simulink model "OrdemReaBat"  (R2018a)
settings: Solver=VariableStepAuto  StartTime=0.0  StopTime=10  RelTol=1e-3
undefined symbols (not defined in the file): bb0aaedc, OrdemReaBat, sdiscope

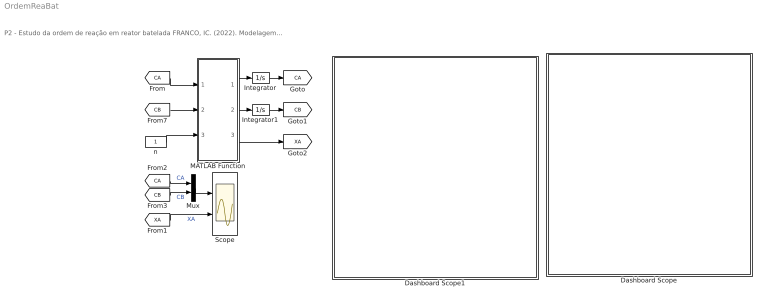
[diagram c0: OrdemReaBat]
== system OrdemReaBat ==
  note: P2 - Estudo da ordem de reação em reator batelada FRANCO, IC. (2022). Modelagem e Simulação: Problemas Típicos da Engenharia Química para Simulação e Análise. NOTAS DE AULA INOVADORAS. The Journal of Engineering and Exact Sciences. Material Complementar.
  Dashboard Scope : Subsystem  DialogController=hmiCreateDDGDialog  IsWebBlock=on  mask(MWDashboardBlock){webBlockId=bb0aaedc-e254-47b2-83d2-97ef23d4ce5b, webBlockType=sdiscope, ShowInitialText=on, HMISrcModelName=OrdemReaBat}
      mask prompts: webBlockId "WebBlock Id"; webBlockType "WebBlock Type"; HMISrcModelName "Source Model"
      mask help: SimulinkHMI:dialogs:HMIScopeDialogDesc
  Dashboard Scope1 : Subsystem  DialogController=hmiCreateDDGDialog  IsWebBlock=on  mask(MWDashboardBlock){webBlockId=9562f2ce-4f72-4572-9857-123cd0054c03, webBlockType=sdiscope, ShowInitialText=on, HMISrcModelName=OrdemReaBat}
      mask prompts: webBlockId "WebBlock Id"; webBlockType "WebBlock Type"; HMISrcModelName "Source Model"
      mask help: SimulinkHMI:dialogs:HMIScopeDialogDesc
  Integrator : Integrator  InitialCondition=1  LowerSaturationLimit=0
  Integrator1 : Integrator  LowerSaturationLimit=0
  MATLAB Function : MATLAB Function  TreatAsAtomicUnit=on
  Mux : Mux  Inputs=2
  Scope : Scope  NumInputPorts=2
  n : Constant
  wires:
  MATLAB Function/1(dCA) -> Integrator/1
  Integrator/1 -> [CA]
  [CA] -> MATLAB Function/1(CA)
  [CA] -> Mux/1  "CA"
  [CB] -> Mux/2  "CB"
  MATLAB Function/3(XA) -> [XA]
  Integrator1/1 -> [CB]
  MATLAB Function/2(dCB) -> Integrator1/1
  [CB] -> MATLAB Function/2(CB)
  n/1 -> MATLAB Function/3(n)
  Mux/1 -> Scope/1
  [XA] -> Scope/2  "XA"

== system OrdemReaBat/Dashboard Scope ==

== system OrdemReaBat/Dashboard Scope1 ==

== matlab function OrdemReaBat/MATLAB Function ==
function [dCA,dCB,XA] = fcn(CA,CB,n)
%% dados do processo
CA0 = 1.00;
k   = 1.30;

%% equações auxiliares
XA=(CA0-CA)/CA0;

%% condicional para evitar concentração negativa
if CA<0
   CA=0;
end

%% modelos matemáticos
dCA = -k*CA^n;
dCB = +k*CA^n;
end
